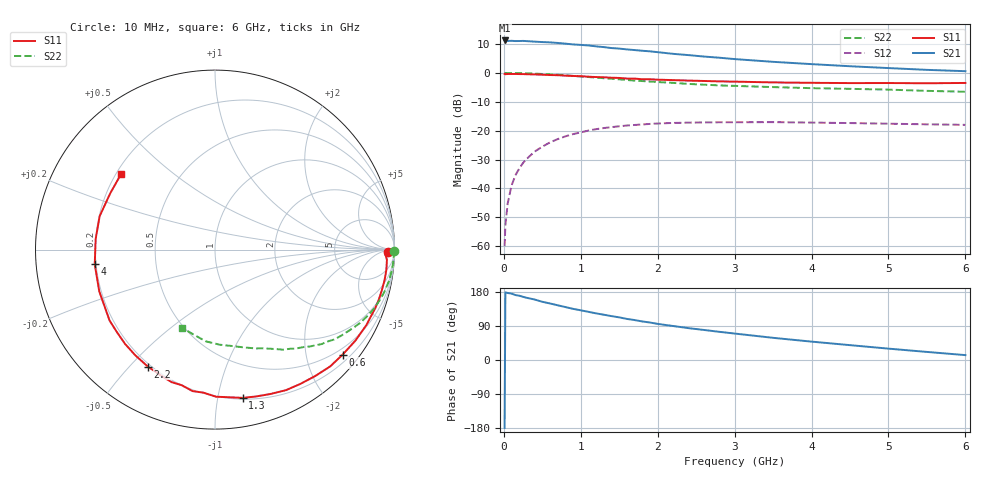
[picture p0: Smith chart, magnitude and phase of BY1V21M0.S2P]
! SIEMENS Small Signal Semiconductors
! BFY420
! Si NPN RF SIEGET Grounded Emitter Transistor in MICRO-X
! VCE = 1.25 V  IC = 1 mA
! Common Emitter S-Parameters:  October  1996
# GHz  S  MA  R  50
!  f  S11  S21  S12  S22
! GHz  MAG  ANG  MAG  ANG  MAG  ANG  MAG  ANG
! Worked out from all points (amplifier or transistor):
!   36 points, 10 MHz to 6 GHz, reference 50 ohm
!   highest |S21| = 11.3 dB at 10 MHz (marker M1)
!   |S21| within 3 dB of that: start of sweep to 1.565 GHz
!   unconditionally stable (mu >= 1): 4.511 GHz to end of sweep
!   at 250 MHz: K = 0.03, MSG = 21.1 dB, |S12| = -31.2 dB
!   at 1.4 GHz: K = 0.22, MSG = 13.7 dB, |S12| = -18.8 dB
!   at 6 GHz: K = 1.35, MAG = 5.8 dB, |S12| = -18.0 dB
!   S11 on the Smith chart (normalised r, x): 10 MHz: 44, -18; 600 MHz: 0.36, -2.74; 1.3 GHz: 0.21, -1.18; 2.2 GHz: 0.19, -0.56; 4 GHz: 0.19, -0.06; 6 GHz: 0.22, +0.34
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0.01  0.9616 -0.9  3.654 -179.3  0.001 96.5  0.9991 -0.3
0.02  0.9497 -1.6  3.62 178.7  0.0023 82.8  0.9999 -0.7
0.05  0.9595 -3.4  3.576 176.8  0.0055 88.3  0.9964 -1.7
0.1  0.9614 -6.7  3.604 175.2  0.0112 85.4  0.9957 -3.5
0.15  0.96 -10.1  3.566 171.4  0.0169 82.8  0.9938 -5.3
0.2  0.957 -13.4  3.571 169.7  0.022 82.8  0.9916 -6.9
0.25  0.9544 -16.8  3.59 166.7  0.0277 79.5  0.9879 -8.7
0.5  0.9324 -32.9  3.427 153.6  0.0529 69.6  0.9596 -17.2
0.6  0.9208 -39.5  3.385 149.2  0.0627 65.7  0.9446 -20.4
0.8  0.899 -51.5  3.218 139.7  0.0798 57.8  0.9085 -26.4
1.1  0.8617 -69.0  2.994 127.1  0.1006 47.9  0.8497 -34.5
1.3  0.8405 -79.4  2.802 119.5  0.1112 41.7  0.8111 -39.1
1.6  0.7996 -94.6  2.558 108.4  0.123 33.5  0.7556 -45.6
1.8  0.7779 -103.8  2.423 101.7  0.1283 29.0  0.724 -49.0
2.2  0.7516 -119.9  2.143 89.7  0.1362 20.6  0.6731 -55.9
2.4  0.7374 -127.1  2.038 84.1  0.1379 17.6  0.6461 -59.0
2.8  0.7139 -140.1  1.837 74.4  0.1399 11.6  0.6086 -64.6
3.5  0.6855 -160.2  1.558 58.5  0.1407 3.7  0.5688 -73.4
4  0.675 -173.0  1.422 48.5  0.1382 -0.4  0.5452 -80.1
4.5  0.6675 174.9  1.307 39.2  0.1355 -4.0  0.5307 -87.1
5.5  0.6626 151.8  1.131 21.3  0.1289 -7.5  0.4896 -103.6
6  0.6713 141.4  1.073 12.9  0.1263 -7.7  0.4722 -113.1
